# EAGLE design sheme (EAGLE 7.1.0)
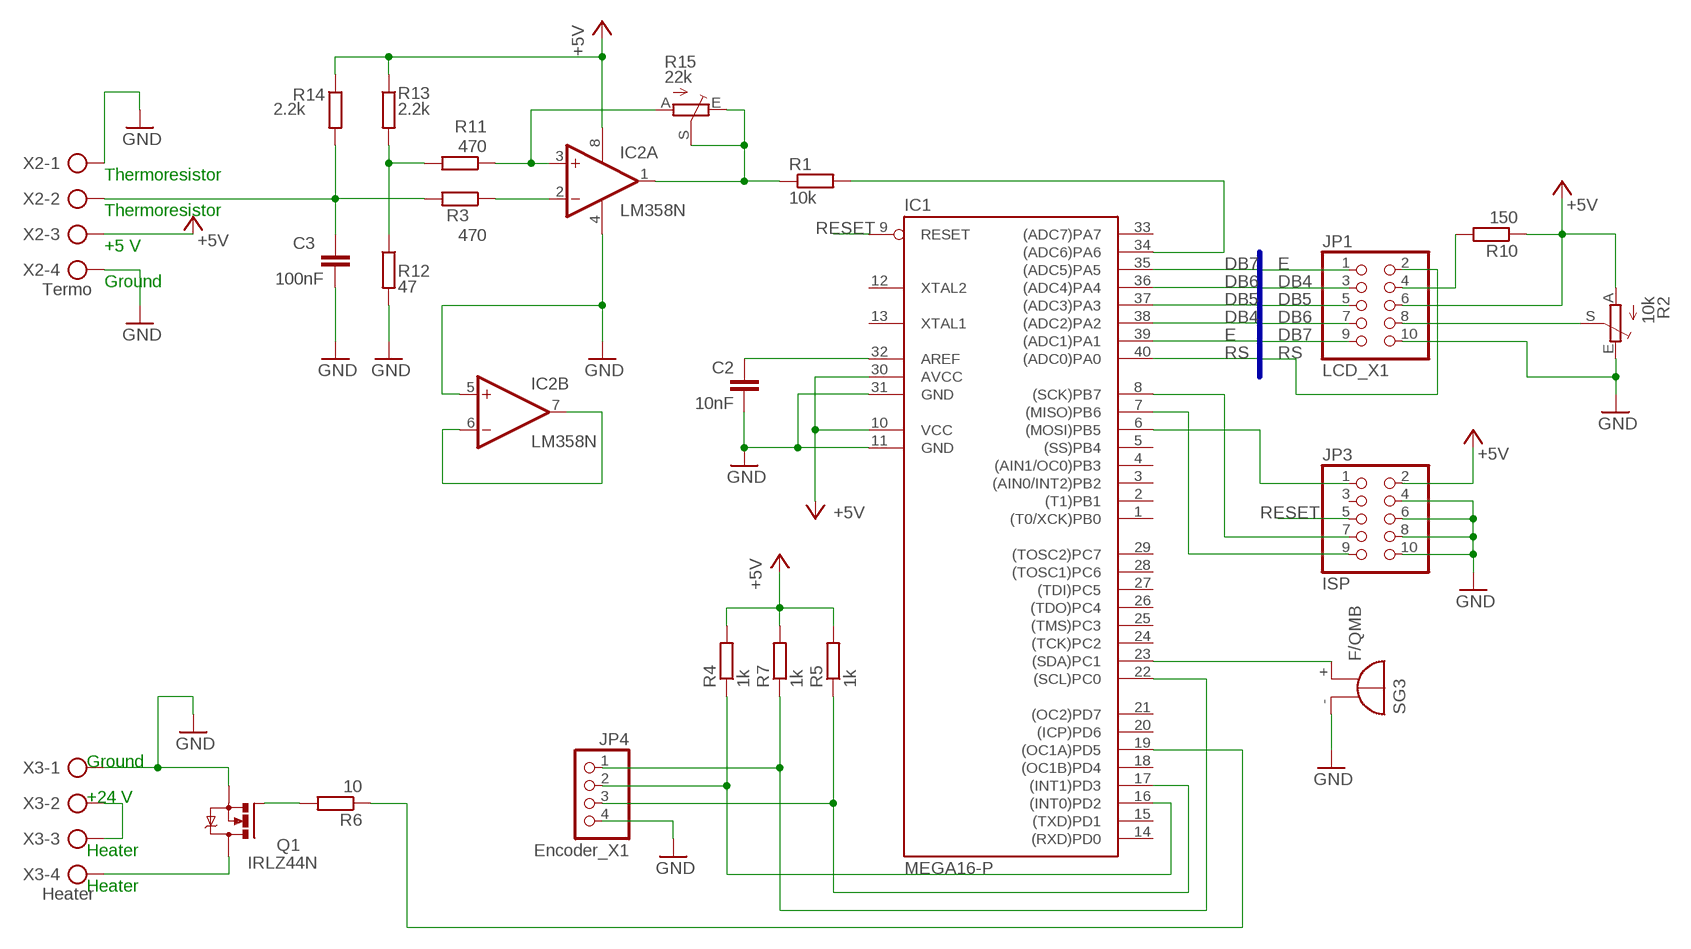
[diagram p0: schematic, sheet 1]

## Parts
C2  10nF  C-EU050-024X044  [C050-024X044]
C3  100nF  C-EU050-024X044  [C050-024X044]
IC1  MEGA16-P  [DIL40]
IC2  LM358N  [DIL08]
JP1  LCD_X1  PINHD-2X5  [2X05]
JP3  ISP  PINHD-2X5  [2X05]
JP4  Encoder_X1  PINHD-1X4  [1X04]
Q1  IRLZ44N  IRLZ44Z  [TO220BH]
R1  10k  R-EU_0207/10  [0207/10]
R2  10k  TRIM_EU-RJ6  [RJ6]
R3  470  R-EU_0207/10  [0207/10]
R4  1k  R-EU_0207/10  [0207/10]
R5  1k  R-EU_0207/10  [0207/10]
R6  10  R-EU_0207/10  [0207/10]
R7  1k  R-EU_0207/10  [0207/10]
R10  150  R-EU_0207/10  [0207/10]
R11  470  R-EU_0207/10  [0207/10]
R12  47  R-EU_0207/10  [0207/10]
R13  2.2k  R-EU_0207/10  [0207/10]
R14  2.2k  R-EU_0207/10  [0207/10]
R15  22k  TRIM_EU-RJ6  [RJ6]
SG3  F/QMB  [F/QMB]
X2  Termo  AK500/4  [AK500/4]
X3  Heater  AK500/4  [AK500/4]

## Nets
+5V: IC1.10(VCC) IC1.30(AVCC) IC2.8(P:V+) JP1.6 JP3.2 R2.A R4.2 R5.2 R7.2 R10.1 R13.1 R14.1 X2.3
DB4: IC1.38((ADC2)PA2) JP1.3
DB5: IC1.37((ADC3)PA3) JP1.5
DB6: IC1.36((ADC4)PA4) JP1.7
DB7: IC1.35((ADC5)PA5) JP1.9
E: IC1.39((ADC1)PA1) JP1.1
GND: C2.2 C3.2 IC1.11(GND) IC1.31(GND) IC2.4(P:V-) IC2.5(B:+IN) JP1.10 JP3.4 JP3.6 JP3.8 JP3.10 JP4.4 Q1.S R2.E R12.2 SG3.-(+) X2.1 X2.4 X3.1
N$1: IC1.23((SDA)PC1) SG3.+(-)
N$2: C2.1 IC1.32(AREF)
N$11: JP1.4 R10.2
N$12: IC1.6((MOSI)PB5) JP3.1
N$13: JP1.8 R2.S
N$14: IC1.7((MISO)PB6) JP3.9
N$15: IC1.8((SCK)PB7) JP3.7
N$16: IC2.3(A:+IN) R11.1 R15.A
N$17: IC1.17((INT1)PD3) JP4.3 R5.1
N$18: IC1.22((SCL)PC0) JP4.1 R7.1
N$19: IC1.16((INT0)PD2) JP4.2 R4.1
N$20: IC1.34((ADC6)PA6) R1.2
N$21: IC2.2(A:-IN) R3.1
N$22: IC2.1(A:OUT) R1.1 R15.E R15.S
N$23: R11.2 R12.1 R13.2
N$24: IC1.19((OC1A)PD5) R6.1
N$25: Q1.G R6.2
N$26: X3.2 X3.3
N$27: C3.1 R3.2 R14.2 X2.2
N$28: Q1.D X3.4
N$29: IC2.6(B:-IN) IC2.7(B:OUT)
RESET: IC1.9(RESET) JP3.5
RS: IC1.40((ADC0)PA0) JP1.2
Unconnected: IC1.1((T0/XCK)PB0) IC1.2((T1)PB1) IC1.3((AIN0/INT2)PB2) IC1.4((AIN1/OC0)PB3) IC1.5((SS)PB4) IC1.12(XTAL2) IC1.13(XTAL1) IC1.14((RXD)PD0) IC1.15((TXD)PD1) IC1.18((OC1B)PD4) IC1.20((ICP)PD6) IC1.21((OC2)PD7) IC1.24((TCK)PC2) IC1.25((TMS)PC3) IC1.26((TDO)PC4) IC1.27((TDI)PC5) IC1.28((TOSC1)PC6) IC1.29((TOSC2)PC7) IC1.33((ADC7)PA7) JP3.3

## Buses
E,DB4,DB5,DB6,DB7,RS

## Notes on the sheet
- Thermoresistor
- Thermoresistor
- +5 V
- Ground
- Ground
- +24 V
- Heater
- Heater

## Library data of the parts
C2 C3 = rcl:C-EU: CAPACITOR, European symbol
IC1 = atmel:MEGA16-P: MICROCONTROLLER 16 Kbytes FLASH 1 kbytes SRAM 512 bytes EEPROM USART 8-channel 10 bit ADC Source: avr.lbr; MPN: ATMEGA16-16PU; OC_FARNELL: 9171142; OC_NEWARK: 01M6885
IC2 = linear:LM358: OP AMP also LM158; LM258; LM2904 Source: http://cache.national.com/ds/LM/LM158.pdf
JP1 JP3 = pinhead:PINHD-2X5: PIN HEADER
JP4 = pinhead:PINHD-1X4: PIN HEADER
Q1 = transistor-power:IRLZ44Z: N-Channel HEXFET® Power MOSFET Logic Level AUTOMOTIVE MOSFET Source: http://www.irf.com/product-info/datasheets/data/irlz44zpbf.pdf
R1 R3-R7 R10-R14 = rcl:R-EU_: RESISTOR, European symbol
R2 R15 = pot:TRIM_EU-: POTENTIOMETER
SG3 = buzzer:F/QMB: BUZZER; OC_FARNELL: unknown; OC_NEWARK: unknown
X2 X3 = con-ptr500:AK500/4: CONNECTOR; OC_FARNELL: unknown; OC_NEWARK: unknown

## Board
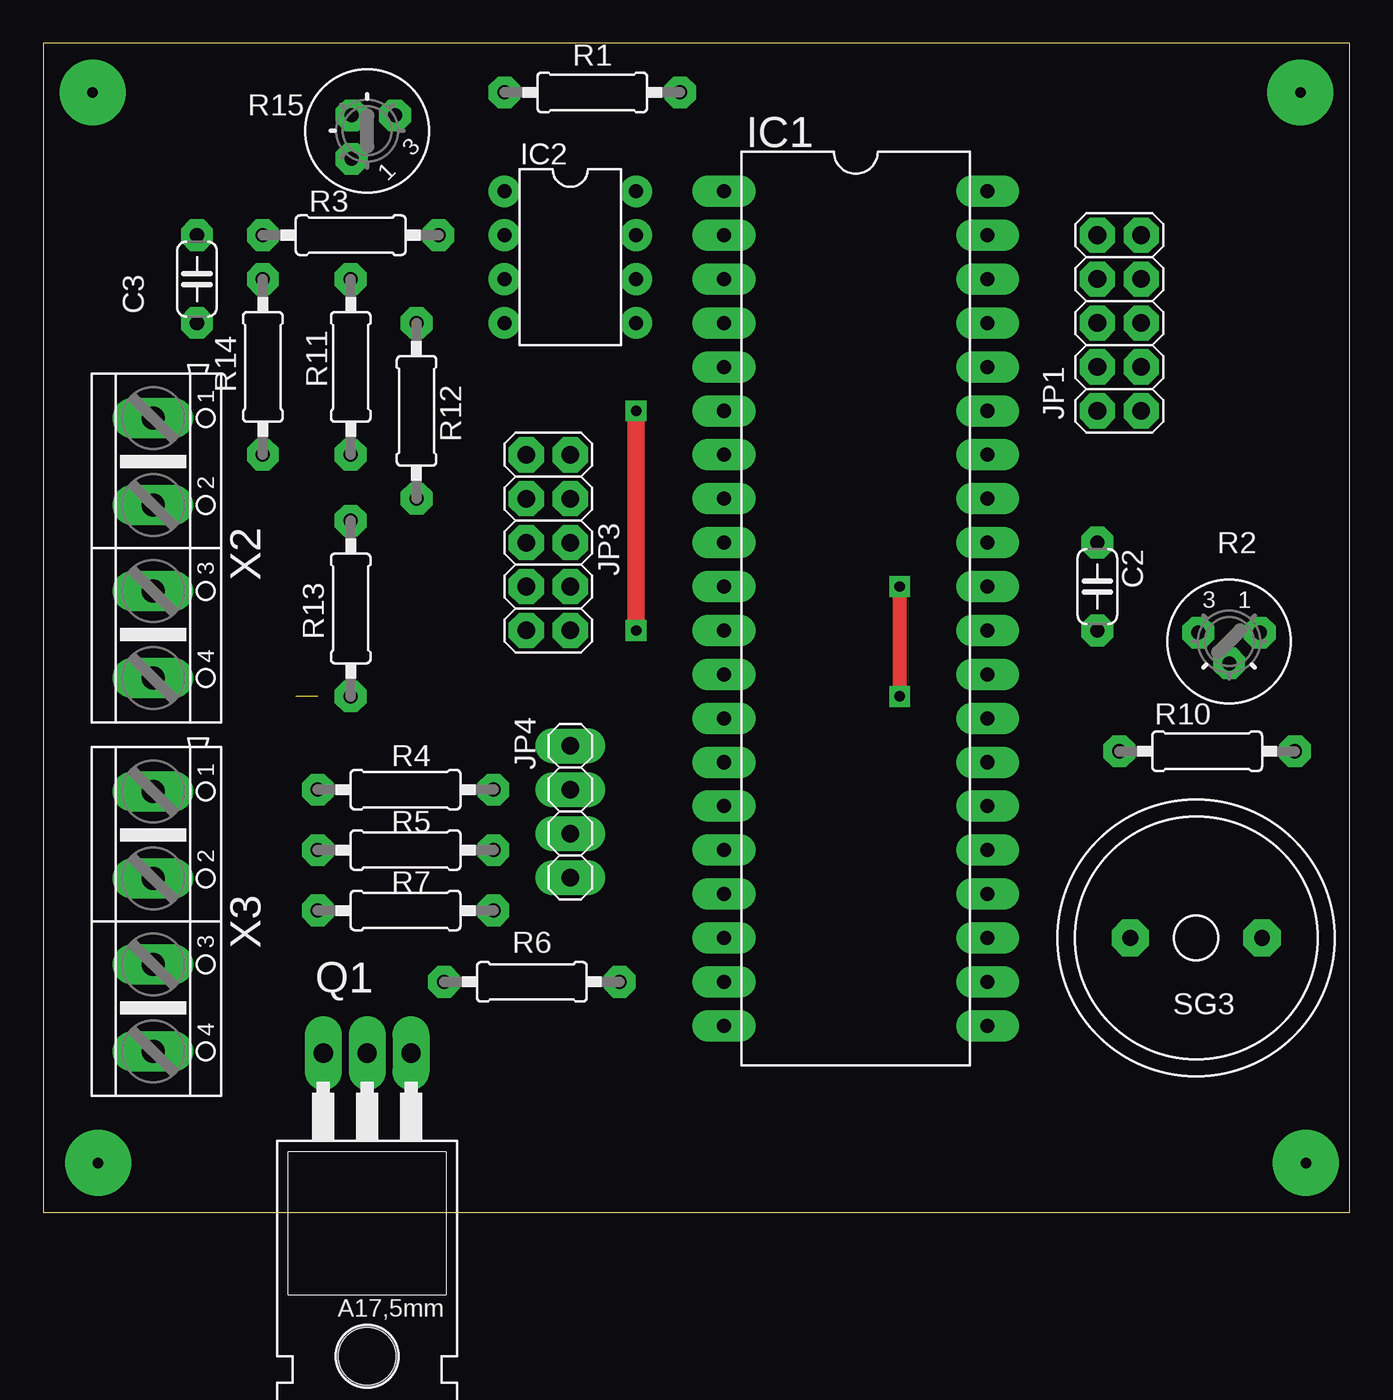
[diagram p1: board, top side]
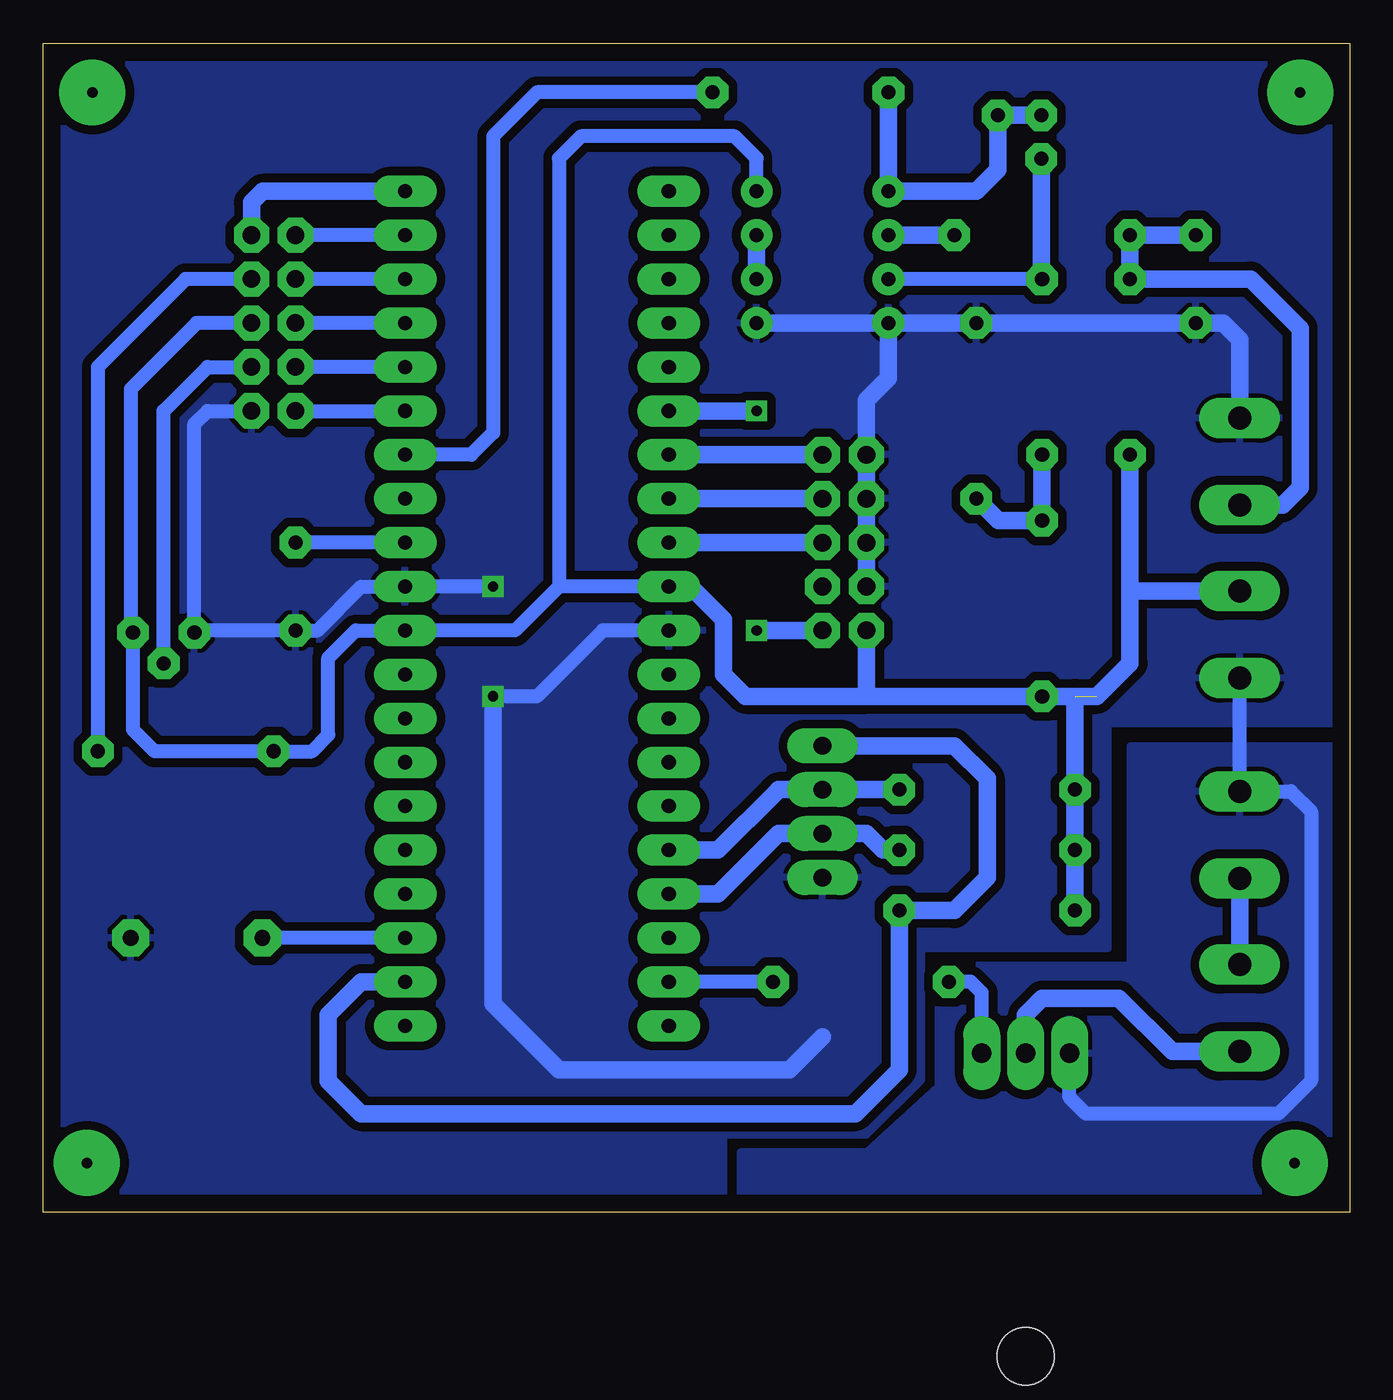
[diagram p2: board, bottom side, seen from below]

Size 75.55 x 67.62 mm. Coordinates in mm from the lower left corner, seen from the top.
Outline: 0,0 75.55,0 75.55,67.62 0,67.62 0,0
Copper layers (1*16): Top 0.035mm / dielectric 1.5mm / Bottom 0.035mm
Design rules "default *": minimum track width 0.3mm, minimum drill 20mil, track to track 20mil, track to pad 12mil, pad to pad 12mil, via to via 12mil, smd to smd 12mil, copper to edge 40mil, drill to drill 20mil, minimum pad ring 20mil, minimum via ring 12mil, stop-mask expansion 4mil, vias tented up to drill 0mil, thermal gap 10mil

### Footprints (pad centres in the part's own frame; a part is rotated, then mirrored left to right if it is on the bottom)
C050-024X044 = drill 0.813 octagon: 1 -2.54,0; 2 2.54,0
DIL40 = drill 0.813 long: 1 -24.13,-7.62; 2 -21.59,-7.62; 3 -19.05,-7.62; 4 -16.51,-7.62; 5 -13.97,-7.62; 6 -11.43,-7.62; 7 -8.89,-7.62; 8 -6.35,-7.62; 9 -3.81,-7.62; 10 -1.27,-7.62; 11 1.27,-7.62; 12 3.81,-7.62; 13 6.35,-7.62; 14 8.89,-7.62; 15 11.43,-7.62; 16 13.97,-7.62; 17 16.51,-7.62; 18 19.05,-7.62; 19 21.59,-7.62; 20 24.13,-7.62; 21 24.13,7.62; 22 21.59,7.62; 23 19.05,7.62; 24 16.51,7.62; 25 13.97,7.62; 26 11.43,7.62; 27 8.89,7.62; 28 6.35,7.62; 29 3.81,7.62; 30 1.27,7.62; 31 -1.27,7.62; 32 -3.81,7.62; 33 -6.35,7.62; 34 -8.89,7.62; 35 -11.43,7.62; 36 -13.97,7.62; 37 -16.51,7.62; 38 -19.05,7.62; 39 -21.59,7.62; 40 -24.13,7.62
DIL08 = drill 0.813 pad 1.27: 1 -3.81,-3.81; 2 -1.27,-3.81; 3 1.27,-3.81; 4 3.81,-3.81; 5 3.81,3.81; 6 1.27,3.81; 7 -1.27,3.81; 8 -3.81,3.81
2X05 = drill 1.016 octagon: 1 -5.08,-1.27; 2 -5.08,1.27; 3 -2.54,-1.27; 4 -2.54,1.27; 5 0,-1.27; 6 0,1.27; 7 2.54,-1.27; 8 2.54,1.27; 9 5.08,-1.27; 10 5.08,1.27
1X04 = drill 1.016 long: 1 -3.81,0; 2 -1.27,0; 3 1.27,0; 4 3.81,0
TO220BH = drill 1.118 long: D 0,-6.35; G -2.54,-6.35; S 2.54,-6.35 | hole 3.302: 0,11.176
0207/10 = drill 0.813 octagon: 1 -5.08,0; 2 5.08,0
RJ6 = drill 0.813 octagon: A -1.778,-0.508; E 1.778,-0.508; S 0,1.27
F/QMB = drill 0.914 pad 2.159 octagon: + 3.81,0; - -3.81,0
AK500/4 = drill 1.321 long: 1 -7.518,0; 2 -2.489,0; 3 2.489,0; 4 7.518,0

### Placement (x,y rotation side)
C2  60.96,36.2 270 top
C3  8.89,53.98 270 top
IC1  46.99,34.92 270 top
IC2  30.48,55.24 270 top
JP1  62.23,51.43 270 top
JP3  29.21,38.74 90 top
JP4  30.48,23.18 270 top
Q1  18.73,2.86 180 top
R1  31.75,64.77 0 top
R2  68.58,33.02 180 top
R3  17.78,56.51 180 top
R4  20.95,24.45 180 top
R5  20.95,20.95 180 top
R6  28.26,13.34 180 top
R7  20.95,17.46 180 top
R10  67.31,26.67 0 top
R11  17.78,48.9 270 top
R12  21.59,46.35 90 top
R13  17.78,34.92 90 top
R14  12.7,48.9 90 top
R15  18.73,62.55 45 top
SG3  66.67,15.88 180 top
X2  6.35,38.42 270 top
X3  6.35,16.83 270 top

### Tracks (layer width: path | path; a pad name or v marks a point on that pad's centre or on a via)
+5V  (1 unrouted)
  Bottom 0.813: JP1.6 66.67,51.43 70.48,47.63 70.48,33.66 R2.A 70.36,27.94 69.09,26.67 R10.1 60.01,26.67 59.05,27.62 59.05,32.07 57.47,33.66 IC1.30 48.26,33.66 45.72,36.2 | IC1.10 45.72,36.2 | IC2.8 34.29,60.96 35.56,62.23 44.45,62.23 45.72,60.96 45.72,36.2
  Bottom 1.016: IC1.10 38.1,36.2 36.19,34.29 36.19,31.12 34.92,29.84 27.94,29.84 | JP3.2 27.94,29.84 | R7.2 R5.2 R4.2 15.88,29.84 | 27.94,29.84 R13.1 14.6,29.84 12.7,31.75 12.7,35.88 | 12.7,35.88 R14.1 | X2.3 12.65,35.93 12.7,35.88
DB4
  Bottom 0.813: IC1.38 JP1.3
DB5
  Bottom 0.813: IC1.37 JP1.5
DB6
  Bottom 0.813: IC1.36 JP1.7
DB7
  Bottom 0.813: JP1.9 IC1.35
E
  Bottom 0.813: IC1.39 JP1.1
GND  (via drill 0.6)
  Top 0.813: v49.53,29.84 v49.53,36.2
  Bottom 0.813: JP1.10 66.04,46.35 66.8,45.59 R2.E 66.67,33.66 C2.2 59.69,33.66 57.15,36.2 IC1.31 v49.53,36.2 | IC1.11 43.18,33.66 46.99,29.84 v49.53,29.84 | Q1.S 16.19,6.67 15.24,5.72 4.13,5.72 2.22,7.62 2.22,23.18 3.39,24.35 X3.1 X2.4
  Bottom 1.016: JP3.4 JP3.6 JP3.8 JP3.10 27.94,46.99 26.67,48.26 IC2.4 | IC2.4 R12.2 C3.2 7.3,51.43 6.35,50.48 X2.1 | v49.53,29.84 49.53,12.06 45.72,8.26 32.38,8.26 30.48,10.16 | IC2.5 IC2.4
  pour Bottom: 75.25,0.64 74.93,66.99 0.63,66.99 0.63,28.26 13.97,28.26 13.97,15.24 24.77,15.24 24.77,7.62 27.94,4.45 36.19,4.45 36.19,0.64
  pour Bottom: 0.63,26.99 12.7,26.99 12.7,14.29 23.81,14.29 23.81,7.3 27.94,3.49 35.24,3.49 35.24,0.64 0.95,0.64
N$1
  Bottom 0.813: IC1.23 SG3.+
N$2
  Bottom 0.813: IC1.32 C2.1
N$7  (via drill 0.6 pad 3.81)
  other vias: 2.86,64.77
N$8  (via drill 0.6 pad 3.81)
  other vias: 3.17,2.86
N$9  (via drill 0.6 pad 3.81)
  other vias: 73.02,2.86
N$10  (via drill 0.6 pad 3.81)
  other vias: 72.71,64.77
N$11
  Bottom 0.813: JP1.4 67.31,53.98 72.39,48.9 R10.2
N$12  (via drill 0.6)
  Top 1.016: v34.29,46.35 v34.29,33.66
  Bottom 1.016: IC1.6 v34.29,46.35 | v34.29,33.66 JP3.1
N$13
  Bottom 0.813: R2.S 68.58,46.35 66.04,48.9 JP1.8
N$14
  Bottom 1.016: JP3.9 IC1.7
N$15
  Bottom 1.016: IC1.8 JP3.7
N$16
  Bottom 0.813: R11.1 IC2.3
  Bottom 1.016: R11.1 17.83,53.98 R15.A
N$17
  Bottom 1.016: R5.1 26.99,20.95 27.94,21.91 JP4.3 33.02,21.91 36.51,18.41 IC1.17
N$18
  Bottom 1.016: IC1.22 57.15,13.34 59.05,11.43 59.05,7.62 57.15,5.72 28.58,5.72 26.03,8.26 R7.1 22.86,17.46 20.95,19.37 20.95,25.08 22.86,26.99 JP4.1
N$19
  Bottom 1.016: IC1.16 36.51,20.95 33.18,24.29 33.02,24.45 JP4.2 R4.1
N$20
  Bottom 0.813: R1.2 46.99,64.77 49.53,62.23 49.53,45.09 50.8,43.82 IC1.34
N$21
  Bottom 1.016: R3.1 IC2.2
N$22
  Bottom 1.016: R1.1 IC2.1 21.59,59.05 20.35,60.3 R15.E R15.S
N$23
  Bottom 1.016: R12.1 20.32,40.01 R13.2 R11.2
N$24
  Bottom 0.813: R6.1 IC1.19
N$25
  Bottom 0.813: Q1.G 21.27,12.7 21.91,13.34 R6.2
N$26
  Bottom 1.016: X3.2 X3.3
N$27
  Bottom 1.016: C3.1 R3.2 R14.2 5.71,53.98 2.86,51.12 2.86,41.91 3.86,40.91 X2.2
N$28
  Bottom 1.016: X3.4 10.26,9.31 13.33,12.38 17.78,12.38 18.73,11.43 Q1.D
N$29
  Bottom 1.016: IC2.6 IC2.7
RESET
  Bottom 1.016: IC1.9 JP3.5
RS
  Bottom 1.016: IC1.40 62.86,59.05 63.5,58.42 JP1.2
